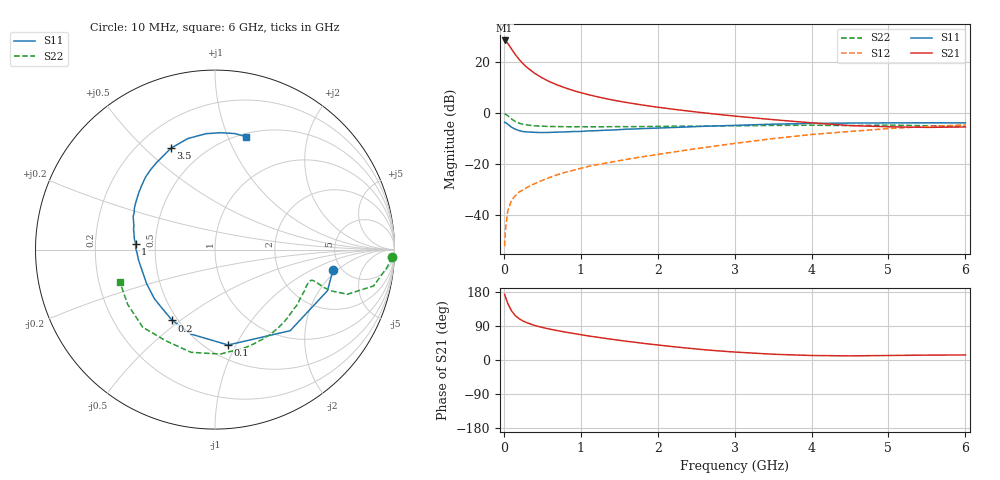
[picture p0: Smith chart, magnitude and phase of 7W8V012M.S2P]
! Infineon Technologies  Discrete & RF Semiconductors
! BFS17W
! Si NPN RF Bipolar Junction Transistor in SOT323
! VCE = 8 V  IC = 12 mA
! Common Emitter S-Parameters:  August  1999
# GHz  S  MA  R  50
!  f  S11  S21  S12  S22
! GHz  MAG  ANG  MAG  ANG  MAG  ANG  MAG  ANG
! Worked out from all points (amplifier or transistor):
!   36 points, 10 MHz to 6 GHz, reference 50 ohm
!   highest |S21| = 28.6 dB at 10 MHz (marker M1)
!   |S21| within 3 dB of that: start of sweep to 92.56 MHz
!   unconditionally stable (mu >= 1): 396.8 MHz to 2.14 GHz; 5.498 GHz to end of sweep
!   at 250 MHz: K = 0.82, MSG = 24.7 dB, |S12| = -30.0 dB
!   at 1.4 GHz: K = 1.16, MAG = 9.8 dB, |S12| = -19.1 dB
!   at 6 GHz: K = 1.03, MAG = -1.5 dB, |S12| = -4.5 dB
!   S11 on the Smith chart (normalised r, x): 10 MHz: 4.25, -1.76; 100 MHz: 0.62, -0.93; 200 MHz: 0.47, -0.47; 1 GHz: 0.39, +0.03; 3.5 GHz: 0.33, +0.60; 6 GHz: 0.53, +1.16
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0.01  0.6672 -9.9  26.96 173.5  0.0025 83.1  0.9896 -2.5
0.02  0.667 -20.1  26.57 166.9  0.0051 91.2  0.9637 -5.9
0.05  0.6161 -47.2  23.82 149.8  0.0121 70.9  0.9065 -12.9
0.1  0.5364 -82.2  18.36 129.7  0.0199 60.2  0.7795 -18.6
0.15  0.4894 -105.8  14.21 116.9  0.0245 57.0  0.6923 -19.5
0.2  0.461 -121.1  11.4 108.8  0.0289 57.5  0.643 -19.2
0.25  0.4397 -132.5  9.417 102.9  0.0316 57.2  0.6115 -18.4
0.3  0.4343 -141.2  8.003 98.3  0.0354 59.1  0.5938 -17.9
0.4  0.4258 -153.4  6.135 91.2  0.042 61.2  0.5712 -17.5
0.5  0.422 -161.5  4.962 85.9  0.0488 63.7  0.5621 -17.7
0.6  0.4249 -167.6  4.154 81.4  0.0559 65.0  0.5553 -18.5
0.7  0.4306 -172.6  3.591 77.4  0.0632 66.2  0.5518 -19.6
0.8  0.4342 -177.2  3.161 73.6  0.0702 67.3  0.5493 -21.1
1  0.4436 175.8  2.552 66.8  0.0842 68.2  0.5495 -24.1
1.1  0.4544 172.0  2.332 63.5  0.0915 69.3  0.5479 -26.2
1.6  0.4923 157.8  1.633 49.3  0.1258 71.1  0.5496 -36.7
2.2  0.5304 143.1  1.211 35.2  0.1748 73.1  0.5605 -51.4
2.8  0.5716 128.9  0.953 23.9  0.2353 72.2  0.5678 -67.4
3.5  0.6161 113.5  0.755 15.2  0.3215 67.8  0.5827 -87.0
4.5  0.6478 94.4  0.578 10.9  0.443 55.8  0.5773 -118.4
5.5  0.6558 80.4  0.533 12.9  0.5538 42.6  0.5743 -148.0
6  0.6529 74.8  0.543 13.3  0.5979 36.1  0.56 -161.4
